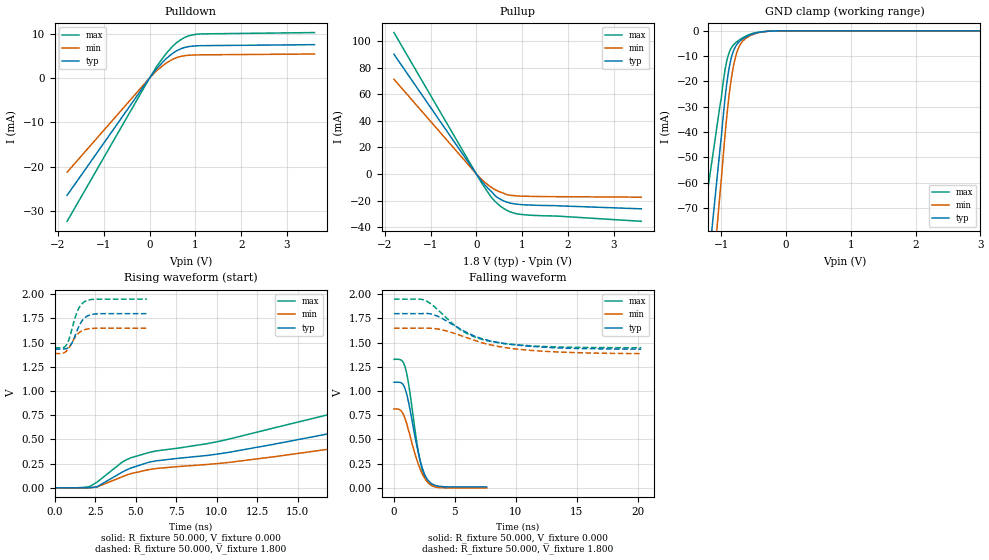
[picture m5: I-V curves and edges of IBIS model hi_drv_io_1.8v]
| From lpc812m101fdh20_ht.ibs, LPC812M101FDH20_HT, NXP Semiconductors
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[Model]   hi_drv_io_1.8v
Model_type I/O
Vinl=5.400E-01
Vinh=1.260E+00
Vref=0.000E+00
Rref=1.000E+06
Cref=2.000E-11
Vmeas=9.000E-01
C_comp   8.440E-13   8.280E-13   8.600E-13
[Voltage Range]   1.800E+00   1.650E+00   1.950E+00
[POWER Clamp Reference]   1.800E+00   1.650E+00   1.950E+00
[GND Clamp Reference]   0.000E+00   0.000E+00   0.000E+00
[Pullup Reference]   1.800E+00   1.650E+00   1.950E+00
[Pulldown Reference]   0.000E+00   0.000E+00   0.000E+00
[Temperature Range]   25   105   -40
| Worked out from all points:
|   slope of the pulldown table from 0 to 0.27 V, typ, clamps not added: 80.1 ohm
|   slope of the pullup table from 0 to 0.27 V, typ, clamps not added: 23.9 ohm
|   GND clamp passes 1 mA (typ) near -0.49 V on its own axis
|   rising waveform, R_fixture 50.000, V_fixture 0.000: 20-80 % time 24.9ns typ, 26.2ns min, 22.6ns max; typ from 0 V to 1.08 V
|   falling waveform, R_fixture 50.000, V_fixture 0.000: 20-80 % time 1.06ns typ, 1.19ns min, 949ps max; typ from 1.09 V to 0.009 V
|   rising waveform, R_fixture 50.000, V_fixture 1.800: 20-80 % time 595ps typ, 618ps min, 564ps max; typ from 1.43 V to 1.8 V
|   falling waveform, R_fixture 50.000, V_fixture 1.800: 20-80 % time 4.05ns typ, 4.73ns min, 3.36ns max; typ from 1.8 V to 1.43 V
[GND Clamp]
-1.8V     -244.7mA   -294.7mA   -167mA
-1.02V    -46.52mA   -64.09mA   -29.35mA
-940mV    -25.93mA   -40.25mA   -14.92mA
-900mV    -17.84mA   -29.88mA   -10.21mA
-860mV    -12.13mA   -21.41mA   -7.428mA
-820mV    -8.42mA    -14.88mA   -5.782mA
-780mV    -6.161mA   -10.21mA   -4.745mA
-740mV    -4.723mA   -7.073mA   -3.919mA
-680mV    -3.339mA   -4.344mA   -2.881mA
-500mV    -1.101mA   -1.317mA   -892.5uA
-240mV    -116.5uA   -126.1uA   -97.57uA
3.6V      0A         0A         0A
[POWER Clamp]
-2.5V     0A         0A         0A
5V        0A         0A         0A
[Pullup]
-1.8V     90.07mA    71.26mA    106.4mA
40mV      -1.925mA   -1.516mA   -2.392mA
180mV     -8.017mA   -6.069mA   -10.14mA
320mV     -12.93mA   -9.85mA    -17.19mA
420mV     -16.61mA   -11.94mA   -20.97mA
540mV     -19.26mA   -13.78mA   -24.54mA
740mV     -21.88mA   -15.96mA   -28.52mA
1.02V     -23.13mA   -16.7mA    -30.55mA
3.6V      -26.18mA   -17.42mA   -35.55mA
[Pulldown]
-1.8V     -26.45mA   -21.25mA   -32.33mA
0V        0A         0A         0A
140mV     1.894mA    1.494mA    2.352mA
320mV     3.921mA    3.039mA    4.945mA
500mV     5.53mA     4.194mA    7.104mA
600mV     6.19mA     4.629mA    8.047mA
740mV     6.8mA      4.988mA    8.997mA
880mV     7.124mA    5.147mA    9.584mA
1.14V     7.298mA    5.229mA    9.953mA
3.6V      7.517mA    5.412mA    10.25mA
[Rising Waveform]
R_fixture = 50.000
V_fixture = 0.000
V_fixture_min = 0.000
V_fixture_max = 0.000
|  time   V(typ)   V(min)   V(max)
0s        0V         0V         0V
2.2ns     1.207mV    1.298mV    17.92mV
4.2ns     165.6mV    116.7mV    270.2mV
5.8ns     263.8mV    188.1mV    364.5mV
10ns      347.7mV    250.1mV    475.6mV
20.2ns    655.5mV    471.7mV    877mV
26.9ns    813.4mV    592.2mV    1.063V
34.3ns    930.5mV    684.7mV    1.188V
44.5ns    1.025V     762.5mV    1.282V
58.8ns    1.083V     815.6mV    1.325V
[Falling Waveform]
R_fixture = 50.000
V_fixture = 0.000
V_fixture_min = 0.000
V_fixture_max = 0.000
|  time   V(typ)   V(min)   V(max)
0s        1.091V     815.6mV    1.328V
500ps     1.09V      805.2mV    1.325V
900ps     1.029V     720.2mV    1.255V
1.2ns     884.4mV    594.6mV    1.075V
1.8ns     481.5mV    320.5mV    535.8mV
2.1ns     307.5mV    210.8mV    307.2mV
2.4ns     177.8mV    127.3mV    154.7mV
2.7ns     95.86mV    69.01mV    72.79mV
3.8ns     15.37mV    2.29mV     5.66mV
7.6ns     9.298mV    0V         4.077mV
[Rising Waveform]
R_fixture = 50.000
V_fixture = 1.800
V_fixture_min = 1.650
V_fixture_max = 1.950
|  time   V(typ)   V(min)   V(max)
0s        1.433V     1.387V     1.448V
500ps     1.434V     1.391V     1.448V
700ps     1.438V     1.41V      1.471V
800ps     1.444V     1.428V     1.501V
1ns       1.477V     1.482V     1.603V
1.4ns     1.634V     1.587V     1.826V
1.6ns     1.704V     1.615V     1.887V
1.9ns     1.763V     1.637V     1.93V
2.6ns     1.798V     1.649V     1.949V
5.7ns     1.8V       1.65V      1.95V
[Falling Waveform]
R_fixture = 50.000
V_fixture = 1.800
V_fixture_min = 1.650
V_fixture_max = 1.950
|  time   V(typ)   V(min)   V(max)
0s        1.8V       1.65V      1.95V
2.1ns     1.8V       1.65V      1.949V
2.6ns     1.801V     1.65V      1.935V
3.6ns     1.772V     1.642V     1.84V
5.5ns     1.638V     1.573V     1.629V
6.6ns     1.569V     1.525V     1.561V
7.8ns     1.522V     1.481V     1.518V
9.4ns     1.485V     1.444V     1.487V
12.1ns    1.455V     1.413V     1.462V
20.3ns    1.433V     1.387V     1.448V
[Ramp]
dV/dt_r   6.4905E-01/2.4968E-08   4.9163E-01/2.6307E-08   7.9413E-01/2.2616E-08
dV/dt_f   2.2020E-01/4.0369E-09   1.5747E-01/4.7266E-09   3.0112E-01/3.3543E-09
R_load = 50
